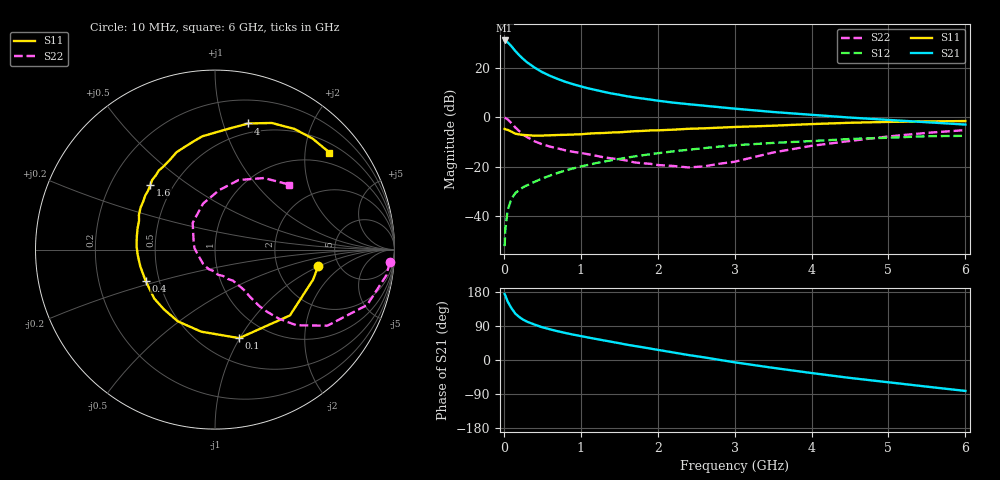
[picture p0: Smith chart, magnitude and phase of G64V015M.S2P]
! SIEMENS Small Signal Semiconductors
! BFG193
! Si NPN RF Bipolar Junction Transistor in SOT223
! VCE = 4 V  IC = 15 mA
! Common Emitter S-Parameters:  August  1996
# GHz  S  MA  R  50
!  f  S11  S21  S12  S22
! GHz  MAG  ANG  MAG  ANG  MAG  ANG  MAG  ANG
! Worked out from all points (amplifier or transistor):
!   36 points, 10 MHz to 6 GHz, reference 50 ohm
!   highest |S21| = 31.0 dB at 10 MHz (marker M1)
!   |S21| within 3 dB of that: start of sweep to 116.1 MHz
!   unconditionally stable (mu >= 1): 767.9 MHz to 2.458 GHz
!   at 250 MHz: K = 0.66, MSG = 25.9 dB, |S12| = -28.3 dB
!   at 1.4 GHz: K = 1.05, MAG = 12.1 dB, |S12| = -17.4 dB
!   at 6 GHz: K = 0.87, MSG = 2.3 dB, |S12| = -7.5 dB
!   S11 on the Smith chart (normalised r, x): 10 MHz: 3.52, -0.95; 100 MHz: 0.74, -0.99; 400 MHz: 0.42, -0.18; 1.6 GHz: 0.37, +0.36; 4 GHz: 0.41, +1.21; 6 GHz: 0.71, +2.55
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0.01  0.5829 -8.8  35.4 174.2  0.0025 88.3  0.976 -4.2
0.02  0.5716 -17.0  34.94 169.7  0.0057 78.2  0.9656 -8.5
0.05  0.5557 -41.3  32.52 154.1  0.0134 72.8  0.9022 -20.0
0.1  0.5113 -74.7  26.91 136.4  0.0229 63.3  0.7561 -34.1
0.15  0.4636 -99.6  21.58 122.3  0.0294 57.1  0.6194 -42.9
0.2  0.4501 -117.4  17.89 113.6  0.034 56.3  0.525 -47.2
0.25  0.4378 -130.6  15.03 106.5  0.0386 55.2  0.4476 -50.2
0.3  0.4347 -141.2  12.91 101.3  0.0421 55.7  0.3992 -51.9
0.4  0.4239 -155.9  10.02 93.4  0.0498 56.4  0.3268 -53.5
0.5  0.4265 -167.2  8.102 86.4  0.058 56.6  0.2834 -54.1
0.6  0.4318 -176.1  6.851 81.0  0.0664 56.9  0.2557 -55.3
0.7  0.4379 177.1  5.917 75.9  0.0752 57.0  0.2346 -57.1
0.9  0.4473 164.6  4.634 67.0  0.0927 55.5  0.2004 -59.8
1.1  0.4666 155.3  3.816 59.3  0.1095 53.5  0.1787 -66.4
1.6  0.509 135.0  2.649 40.4  0.1532 45.6  0.133 -87.1
2.2  0.5603 116.5  1.97 20.0  0.2046 34.1  0.1039 -129.4
2.8  0.6158 100.9  1.596 0.5  0.2552 21.3  0.115 175.4
3.5  0.6743 84.3  1.275 -20.7  0.3031 4.9  0.194 129.9
4  0.7269 75.2  1.119 -34.4  0.3303 -4.7  0.2647 104.6
4.5  0.7729 65.9  0.984 -47.3  0.3637 -15.0  0.3321 86.0
5.5  0.8233 48.8  0.792 -70.3  0.4142 -38.6  0.4833 55.6
6  0.8362 40.3  0.711 -81.6  0.4214 -52.4  0.5498 41.2
